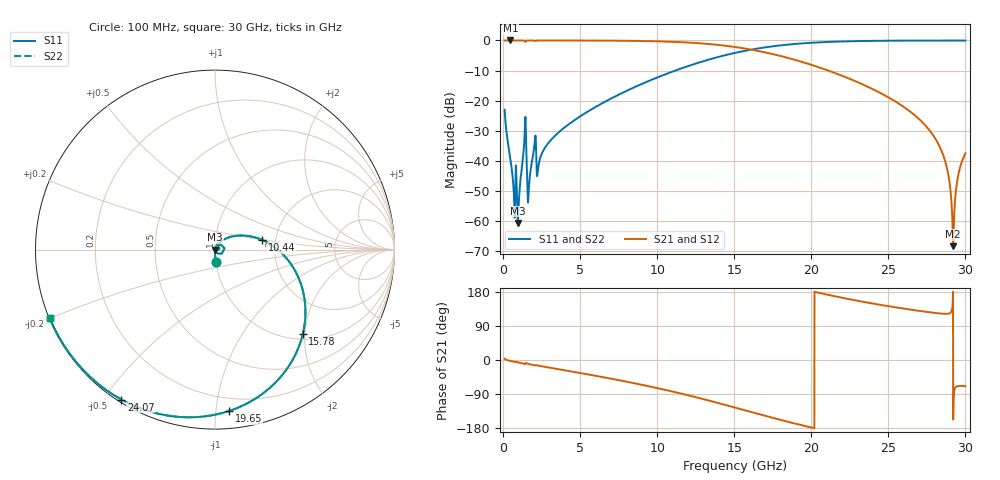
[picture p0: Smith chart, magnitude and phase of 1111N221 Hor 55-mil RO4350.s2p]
# GHz S MA R 50
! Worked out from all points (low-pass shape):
!   3201 points, 100 MHz to 30 GHz, reference 50 ohm
!   highest |S21| = 0.00 dB at 473.8 MHz (marker M1); lowest = -68.3 dB at 29.21 GHz (marker M2)
!   |S21| within 3 dB of the highest: start of sweep to 16.06 GHz
!   lowest |S11| = -60.6 dB at 959.6 MHz (marker M3), VSWR 1.00, Z = 50.1 - j0.00261 ohm
!   |S11| at or under -10 dB: start of sweep to 11.17 GHz
!   |S22| runs from -60.6 to 0.0 dB; largest |S21 - S12| = 0
!   S11 on the Smith chart (normalised r, x): 100 MHz: 1.00, -0.14; 10.44 GHz: 1.70, +0.20; 15.78 GHz: 1.11, -1.95; 19.65 GHz: 0.11, -1.08; 24.07 GHz: 0.01, -0.55; 30 GHz: 0.00, -0.20
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0.1  0.07087 -86.4  0.9973 3.4  0.9973 3.4  0.07087 -86.4
0.47375  0.01079 -90.5  0.9995 -2.4  0.9995 -2.4  0.01079 -90.5
0.6419375  0.004746 -88.3  0.9995 -3.8  0.9995 -3.8  0.004746 -88.3
0.959625  0.0009319 -1.6  0.999 -6.1  0.999 -6.1  0.0009319 -1.6
1.37075  0.01993 67.4  0.9952 -9.8  0.9952 -9.8  0.01993 67.4
1.688438  0.003982 58.2  0.9984 -10.9  0.9984 -10.9  0.003982 58.2
1.996781  0.01514 66.2  0.9969 -13.5  0.9969 -13.5  0.01514 66.2
2.314469  0.008781 63.5  0.998 -15.1  0.998 -15.1  0.008781 63.5
5.089563  0.05686 54.1  0.9968 -34.9  0.9968 -34.9  0.05686 54.1
10.06978  0.2466 14.8  0.9662 -74.7  0.9662 -74.7  0.2466 14.8
10.44353  0.269 11.5  0.9601 -78.1  0.9601 -78.1  0.269 11.5
15.05  0.6213 -35.8  0.7783 -125.5  0.7783 -125.5  0.6213 -35.8
15.77881  0.6793 -44.0  0.7281 -133.7  0.7281 -133.7  0.6793 -44.0
19.64712  0.9026 -85.0  0.4208 -174.7  0.4208 -174.7  0.9026 -85.0
20.03956  0.9159 -88.8  0.3911 -178.5  0.3911 -178.5  0.9159 -88.8
24.06672  0.9847 -122.0  0.1522 148.4  0.1522 148.4  0.9847 -122.0
25.01978  0.99 -128.6  0.1131 141.9  0.1131 141.9  0.99 -128.6
28.17797  0.9963 -147.9  0.0206 123.5  0.0206 123.5  0.9963 -147.9
28.804  0.9965 -151.3  0.007619 121.9  0.007619 121.9  0.9965 -151.3
29.20578  0.9965 -153.5  0.0003854 -157.2  0.0003854 -157.2  0.9965 -153.5
29.56084  0.9965 -155.3  0.00623 -68.6  0.00623 -68.6  0.9965 -155.3
30  0.9964 -157.6  0.01339 -69.0  0.01339 -69.0  0.9964 -157.6
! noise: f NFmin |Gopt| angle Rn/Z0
0.1  0.0006321  0.7223  0.8524  0.0004512
3.417  0.007991  0.3971  20.75  0.002075
6.743  0.01351  0.3408  37.78  0.002913
10.06  0.02026  0.3601  51.91  0.004219
13.39  0.02993  0.431  65.53  0.00653
16.7  0.0462  0.5494  81.31  0.01118
20.03  0.07911  0.6965  100.1  0.02196
23.35  0.162  0.8366  120.2  0.05338
26.67  0.508  0.9439  139.7  0.2422
30  2.227  0.9863  157.6  1.469
